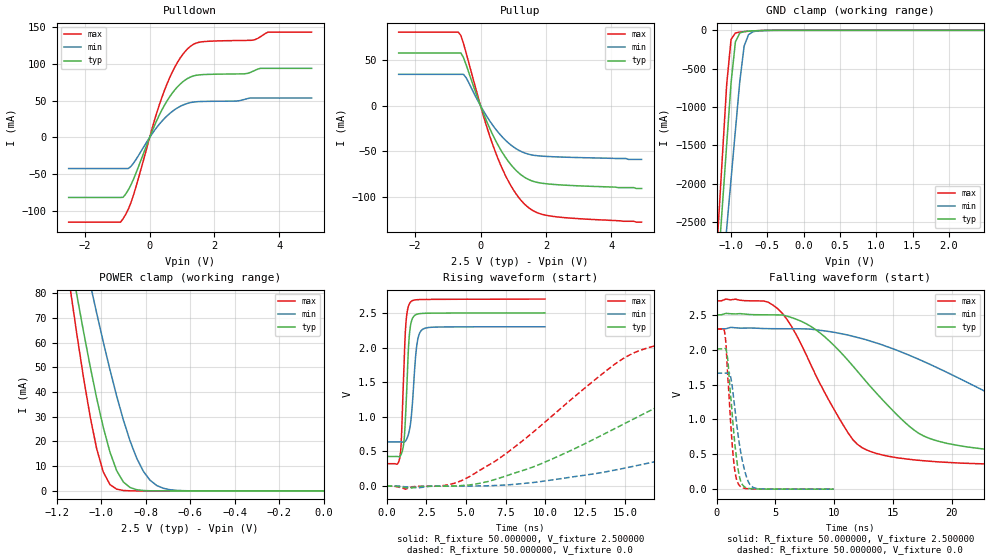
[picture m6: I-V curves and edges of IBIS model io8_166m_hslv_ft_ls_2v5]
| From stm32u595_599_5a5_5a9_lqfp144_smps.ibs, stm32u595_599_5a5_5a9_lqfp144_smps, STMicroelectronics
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|   Model io8_166m_hslv_ft_ls_2v5
[Model]  io8_166m_hslv_ft_ls_2v5
Model_type I/O
Polarity   Non-Inverting
Enable   Active-Low
Vinl =   0.750000V
Vinh =   1.750000V
Vmeas =  1.250000V
Cref =   50.000000pF
Rref =   100.000000M
Vref =   0.0V
C_comp   3.458600pF   3.457900pF   3.495500pF
[Temperature Range]   25.000000   0.140000k   -40.000000
[Pullup Reference]   2.500000V   2.300000V   2.700000V
[Pulldown Reference]   0.0V   0.0V   0.0V
[POWER Clamp Reference]   2.500000V   2.300000V   2.700000V
[GND Clamp Reference]   0.0V   0.0V   0.0V
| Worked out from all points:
|   slope of the pulldown table from 0 to 0.375 V, typ, clamps not added: 10.1 ohm
|   slope of the pullup table from 0 to 0.375 V, typ, clamps not added: 11.7 ohm
|   GND clamp passes 1 mA (typ) near -0.50 V on its own axis
|   POWER clamp passes 1 mA (typ) near -0.86 V on its own axis
|   rising waveform, R_fixture 50.000000, V_fixture 2.500000: 20-80 % time 247ps typ, 328ps min, 231ps max; typ from 0.428 V to 2.5 V
|   rising waveform, R_fixture 50.000000, V_fixture 0.0: 20-80 % time 11.1ns typ, 19.9ns min, 7.41ns max; typ from 0 V to 2.01 V
|   falling waveform, R_fixture 50.000000, V_fixture 2.500000: 20-80 % time 7.02ns typ, 13.9ns min, 4.48ns max; typ from 2.5 V to 0.428 V
|   falling waveform, R_fixture 50.000000, V_fixture 0.0: 20-80 % time 658ps typ, 861ps min, 542ps max; typ from 2.01 V to 0 V
[Pulldown]
|Voltage   I(typ)   I(min)   I(max)
-2.5V     -81.62mA   -42.31mA   -115.3mA
-900mV    -81.62mA   -42.31mA   -115.3mA
-820mV    -81.43mA   -42.31mA   -110.6mA
-500mV    -56.95mA   -35.08mA   -78.57mA
140mV     15.18mA    9.02mA     22.02mA
460mV     44mA       25.98mA    64.38mA
860mV     68.91mA    40.27mA    102.2mA
1.26V     82.21mA    47.42mA    124mA
1.66V     85.54mA    48.99mA    130.3mA
3.18V     89.84mA    53.64mA    132.3mA
3.66V     94.01mA    53.64mA    143.3mA
5V        94.01mA    53.64mA    143.3mA
[Pullup]
|Voltage   I(typ)   I(min)   I(max)
-2.5V     57.98mA    34.47mA    80.92mA
-680mV    57.98mA    34.47mA    80.92mA
-600mV    57.98mA    34.47mA    77.15mA
-440mV    45.11mA    30.85mA    58.07mA
120mV     -11.18mA   -7.509mA   -14.95mA
520mV     -42.31mA   -28.36mA   -56.92mA
760mV     -56.64mA   -37.85mA   -76.55mA
1V        -67.83mA   -45.14mA   -92.22mA
1.48V     -81.29mA   -53.4mA    -112.4mA
1.8V      -84.73mA   -55.19mA   -118.5mA
2.28V     -86.63mA   -56.16mA   -121.9mA
4.92V     -91mA      -59mA      -128mA
[GND_clamp]
|Voltage   I(typ)   I(min)   I(max)
-2.5V     -9.641A    -9.693A    -9.352A
-1.18V    -3.114A    -3.874A    -2.614A
-1.12V    -2.301A    -3.23A     -1.656A
-1.06V    -1.489A    -2.587A    -706.2mA
-1V       -685.8mA   -1.945A    -119.3mA
-940mV    -149.7mA   -1.304A    -34.73mA
-880mV    -35.54mA   -672.6mA   -23.06mA
-820mV    -16.2mA    -206.4mA   -17.27mA
-760mV    -10.58mA   -57.55mA   -12.41mA
-700mV    -7.152mA   -18.74mA   -8.24mA
-400mV    -103.3uA   -378.6uA   -41.75uA
2.48V     0A         13.22nA    0A
[POWER_clamp]
|Voltage   I(typ)   I(min)   I(max)
-2.49V    881mA      773.1mA    1.07A
-1.14V    95.25mA    122.7mA    82.82mA
-1.11V    79.9mA     109.7mA    64.14mA
-1.05V    50.87mA    84.26mA    30.57mA
-1.02V    37.63mA    72.04mA    17.17mA
-990mV    25.71mA    60.25mA    7.621mA
-930mV    8.217mA    38.43mA    713.9uA
-900mV    3.624mA    28.77mA    182.8uA
-840mV    490.7uA    13.24mA    11.35uA
-780mV    56.55uA    4.324mA    699nA
-660mV    716.7nA    226uA      9.784nA
0V        0A         19.53nA    0A
[Ramp]
| variable   typ   min   max
dV/dt_r  1.20666/11.05042n   0.99780/19.92762n   1.37784/7.40096n
dV/dt_f  1.24345/7.00049n   0.99748/13.85698n   1.42637/4.47503n
R_load = 50.000000
[Rising Waveform]
R_fixture= 50.000000
V_fixture= 2.500000
V_fixture_min= 2.300000
V_fixture_max= 2.700000
|time   V(typ)   V(min)   V(max)
0s        427.6mV    637.5mV    322.7mV
840.8ps   428.3mV    637.5mV    415.9mV
940.9ps   468.6mV    637.1mV    715.7mV
1.101ns   655.6mV    635.2mV    1.738V
1.201ns   1.031V     652.3mV    2.287V
1.381ns   1.993V     750.5mV    2.6V
1.522ns   2.333V     922.7mV    2.66V
1.902ns   2.48V      2.025V     2.69V
2.262ns   2.493V     2.261V     2.694V
9.97ns    2.5V       2.3V       2.7V
[Rising Waveform]
R_fixture= 50.000000
V_fixture= 0.0
V_fixture_min= 0.0
V_fixture_max= 0.0
|time   V(typ)   V(min)   V(max)
0s        2.134nV    120.5nV    2.162nV
3.604ns   -1.322mV   -1.026mV   7.164mV
5.205ns   15.24mV    157.2uV    135.3mV
9.61ns    310.7mV    61.83mV    852.3mV
15.62ns   976.5mV    289.2mV    1.929V
20.42ns   1.506V     536mV      2.16V
23.62ns   1.726V     710.7mV    2.218V
37.64ns   1.961V     1.366V     2.288V
56.46ns   2.005V     1.591V     2.296V
199.4ns   2.011V     1.663V     2.296V
[Falling Waveform]
R_fixture= 50.000000
V_fixture= 2.500000
V_fixture_min= 2.300000
V_fixture_max= 2.700000
|time   V(typ)   V(min)   V(max)
0s        2.5V       2.3V       2.7V
4.404ns   2.5V       2.302V     2.681V
6.006ns   2.481V     2.3V       2.432V
7.608ns   2.375V     2.298V     1.937V
12.01ns   1.686V     2.175V     639.8mV
16.42ns   900.3mV    1.919V     428.1mV
18.82ns   690.6mV    1.739V     391.8mV
29.23ns   501mV      983mV      339.3mV
44.84ns   446.6mV    744.5mV    325.5mV
199.4ns   427.6mV    637.5mV    322.7mV
[Falling Waveform]
R_fixture= 50.000000
V_fixture= 0.0
V_fixture_min= 0.0
V_fixture_max= 0.0
|time   V(typ)   V(min)   V(max)
0s        2.011V     1.663V     2.296V
620.6ps   2.011V     1.663V     2.297V
780.8ps   2.014V     1.663V     2.123V
880.9ps   1.946V     1.663V     1.849V
1.161ns   1.412V     1.638V     1.064V
1.461ns   820.6mV    1.297V     398.8mV
1.922ns   203mV      672.8mV    59.04mV
2.482ns   23.66mV    212.7mV    9.459mV
3.083ns   4.525mV    28.17mV    3.596mV
9.97ns    2.134nV    120.5nV    2.162nV
